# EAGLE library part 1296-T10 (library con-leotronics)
1.27mm SINGLE ROW FEMALE SOCKET Source: http://www.leotronics.co.uk/Conexcon/Data%20Sheets/sec.%20A/1296ing.pdf
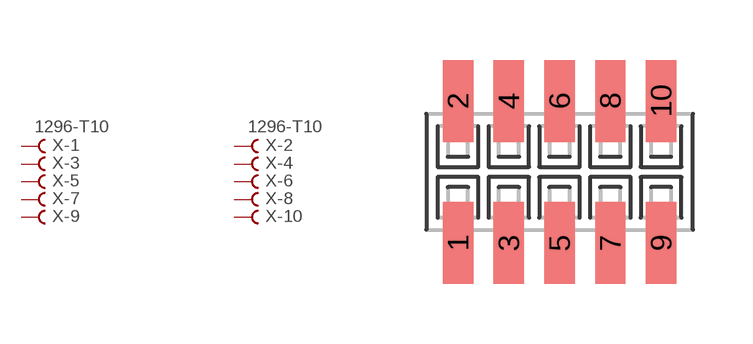
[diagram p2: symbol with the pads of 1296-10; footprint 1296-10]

Designator prefix X; gates -1=FVAL -2=FVAL -3=F -4=F -5=F -6=F -7=F -8=F -9=F -10=F

## 1296-T10 (OC_FARNELL: unknown; OC_NEWARK: unknown)  [1296-10]
1  -1:B  pas
2  -2:B  pas
3  -3:B  pas
4  -4:B  pas
5  -5:B  pas
6  -6:B  pas
7  -7:B  pas
8  -8:B  pas
9  -9:B  pas
10  -10:B  pas

## Footprint 1296-10 (pad centres in mm)
1.27mm SINGLE ROW FEMALE SOCKET Source: http://www.leotronics.co.uk/Conexcon/Data%20Sheets/sec.%20A/1296ing.pdf
smd 0.76 x 2.05: 1 -2.54,-1.78; 2 -2.54,1.78; 3 -1.27,-1.78; 4 -1.27,1.78; 5 0,-1.78; 6 0,1.78; 7 1.27,-1.78; 8 1.27,1.78; 9 2.54,-1.78; 10 2.54,1.78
